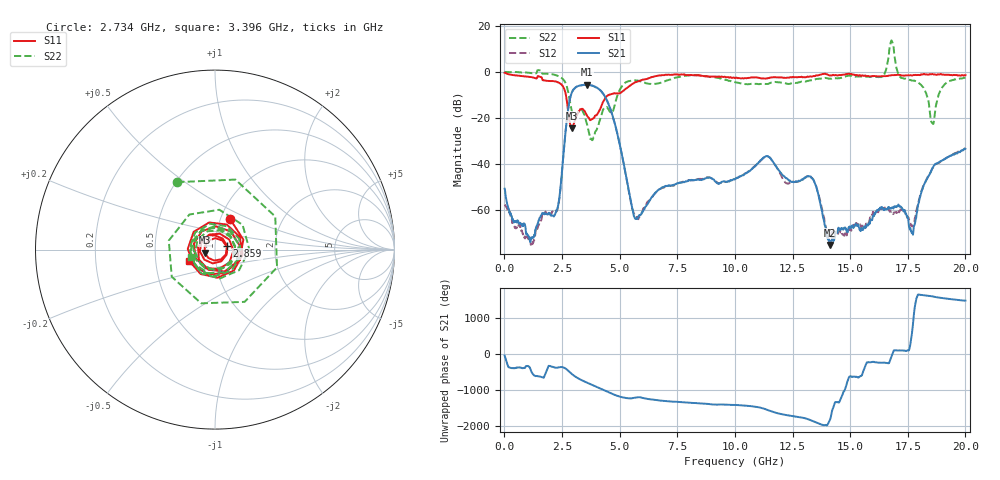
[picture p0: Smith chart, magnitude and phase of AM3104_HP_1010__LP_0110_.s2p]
!Created with skrf (http://scikit-rf.org).
# Hz S RI R 50.0
!freq ReS11 ImS11 ReS21 ImS21 ReS12 ImS12 ReS22 ImS22
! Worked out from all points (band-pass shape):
!   1601 points, 10 MHz to 20 GHz, reference 50 ohm
!   highest |S21| = -5.58 dB at 3.571 GHz (marker M1); lowest = -75.2 dB at 14.14 GHz (marker M2)
!   |S21| within 3 dB of the highest: 2.945 GHz to 4.215 GHz (1.27 GHz wide, 35.5 % of centre)
!   lowest |S11| = -24.5 dB at 2.921 GHz (marker M3), VSWR 1.13, Z = 44.6 - j1.55 ohm
!   |S11| at or under -10 dB: 2.668 GHz to 4.531 GHz (1.863 GHz wide, 51.8 % of centre)
!   |S22| runs from -29.7 to 13.6 dB; largest |S21 - S12| = 0.029
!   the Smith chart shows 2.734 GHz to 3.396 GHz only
!   S11 on the Smith chart (normalised r, x): 2.734 GHz: 1.11, +0.39; 2.859 GHz: 1.14, +0.05; 3.396 GHz: 0.74, -0.10
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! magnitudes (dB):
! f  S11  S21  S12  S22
! 10 MHz  -0.4  -50.8  -58.0  0.0
! 1.134 GHz  -2.2  -73.2  -73.9  -0.5
! 2.171 GHz  -4.1  -62.4  -60.8  -1.3
! 2.371 GHz  -4.7  -55.7  -56.2  -2.0
! 2.734 GHz  -14.4  -18.7  -18.7  -7.3
! 2.859 GHz  -23.0  -11.1  -11.2  -13.7
! 2.921 GHz  -24.5  -9.1  -9.2  -16.8
! 3.346 GHz  -16.1  -5.8  -5.9  -16.6
! 3.396 GHz  -16.1  -5.7  -5.8  -17.0
! 3.571 GHz  -18.7  -5.6  -5.7  -22.2
! 4.583 GHz  -9.9  -15.6  -15.8  -17.4
! 5.682 GHz  -4.5  -63.8  -62.5  -3.7
! 6.682 GHz  -1.6  -51.3  -51.4  -5.0
! 10.01 GHz  -2.7  -46.7  -46.5  -4.5
! 11.38 GHz  -2.9  -36.7  -36.8  -5.3
! 13.34 GHz  -2.1  -46.2  -46.0  -3.6
! 14.14 GHz  -1.6  -75.2  -72.7  -3.0
! 16.68 GHz  -1.6  -59.0  -59.9  7.2
! 17.69 GHz  -1.6  -69.9  -66.8  -3.8
! 18.56 GHz  -0.9  -41.9  -42.1  -22.3
! 19.03 GHz  -1.2  -38.3  -38.3  -6.3
! 20 GHz  -1.4  -33.5  -33.2  -2.5
